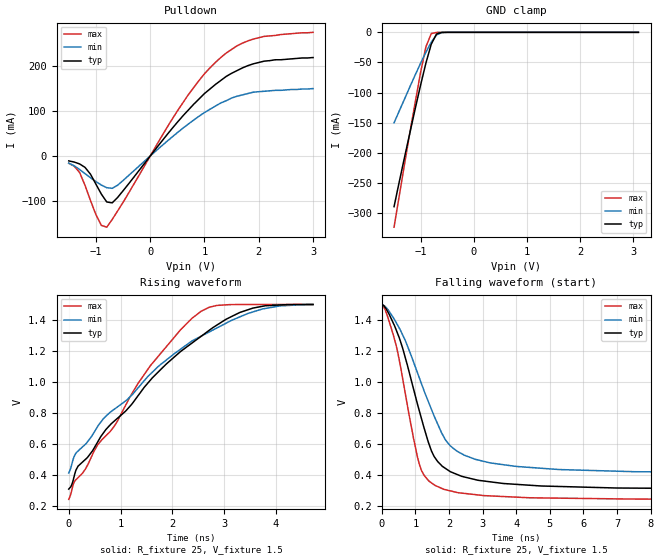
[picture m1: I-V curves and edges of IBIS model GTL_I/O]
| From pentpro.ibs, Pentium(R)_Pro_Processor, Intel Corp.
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[Model]   GTL_I/O
Model_type  I/O_open_drain
Polarity   Inverting
Enable   Active-Low
Vinl = 0.8
Vinh = 1.2
Vmeas = 1.00
Cref  = 0.00p
Rref  = 25.00
Vref  = 1.50
|Variable   typ   min   max
C_comp   3.0p   2.7p   3.3p
|Variable   typ   min   max
[Voltage range] 3.1   2.845   3.255
|Variable   typ   min   max
[Temperature Range] 80   0   100
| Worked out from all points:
|   slope of the pulldown table from 0 to 0.465 V, typ, clamps not added: 6.63 ohm
|   GND clamp passes 1 mA (typ) near -0.63 V on its own axis
|   rising waveform, R_fixture 25, V_fixture 1.5: 20-80 % time 1.98ns typ, 2.08ns min, 1.53ns max; typ from 0.31 V to 1.5 V
|   falling waveform, R_fixture 25, V_fixture 1.5: 20-80 % time 938ps typ, 1.22ns min, 675ps max; typ from 1.5 V to 0.311 V
[Pulldown]
|Volts   typ   min   max
-1.5V     -10.7mA    -15.7mA    -16.1mA
-1.3V     -17.5mA    -29.8mA    -36.5mA
-1.2V     -25.2mA    -39mA      -65.1mA
-900mV    -84.5mA    -64.4mA    -154mA
-800mV    -102mA     -70.3mA    -158mA
-700mV    -104mA     -71.7mA    -141mA
-600mV    -92mA      -64.8mA    -122mA
500mV     75.1mA     52mA       100mA
1.2V      159mA      111mA      208mA
1.6V      190mA      133mA      245mA
1.9V      205mA      142mA      260mA
3V        219mA      150mA      275mA
[Pullup]
|Volts   typ   min   max
-1.5V     0A         0A         0A
3V        0A         0A         0A
[GND_clamp]
|Volts   typ   min   max
-1.5V     -289mA     -150mA     -323mA
-1.3V     -206mA     -110mA     -217mA
-1.2V     -166mA     -89.9mA    -165mA
-1V       -87.3mA    -51.2mA    -66.2mA
-900mV    -50.9mA    -32.9mA    -23.9mA
-800mV    -19.7mA    -16.4mA    -2.14mA
-700mV    -2.72mA    -4.27mA    -134uA
-600mV    -187uA     -406uA     -8.1uA
3.1V      0A         0A         0A
[POWER_clamp]
|Volts   typ   min   max
-600mV    0A         0A         0A
0V        0A         0A         0A
[Ramp]
|Variable   typ   min   max
dV/dt_r   0.71/2.62n 0.65/2.83n 0.75/1.98n
dV/dt_f   0.71/6.74n 0.65/8.80n 0.75/5.40n
[Rising Waveform]
R_fixture = 25
V_fixture = 1.5
C_fixture = 0.00pF
|Time   Typ(v)   Min(v)   Max(v)
0s        310mV      414mV      244mV
60ps      340mV      NA         NA
140ps     433mV      543mV      NA
720ps     695mV      NA         NA
1.46ns    967mV      NA         NA
2.16ns    1.197V     NA         1.337V
2.78ns    1.35V      NA         NA
3.3ns     1.448V     NA         1.5V
3.8ns     1.492V     NA         1.5V
4.72ns    1.5V       1.5V       1.5V
[Falling Waveform]
R_fixture = 25
V_fixture = 1.5
C_fixture = 0.00pF
|Time   Typ(v)   Min(v)   Max(v)
0s        1.5V       1.5V       1.5V
380ps     1.362V     NA         NA
1.06ns    858mV      NA         517mV
1.24ns    717mV      NA         NA
1.48ns    554mV      NA         NA
1.8ns     457mV      NA         NA
2.04ns    422mV      588mV      NA
2.86ns    367mV      NA         NA
4.74ns    330mV      NA         NA
14.66ns   311mV      414mV      244mV
